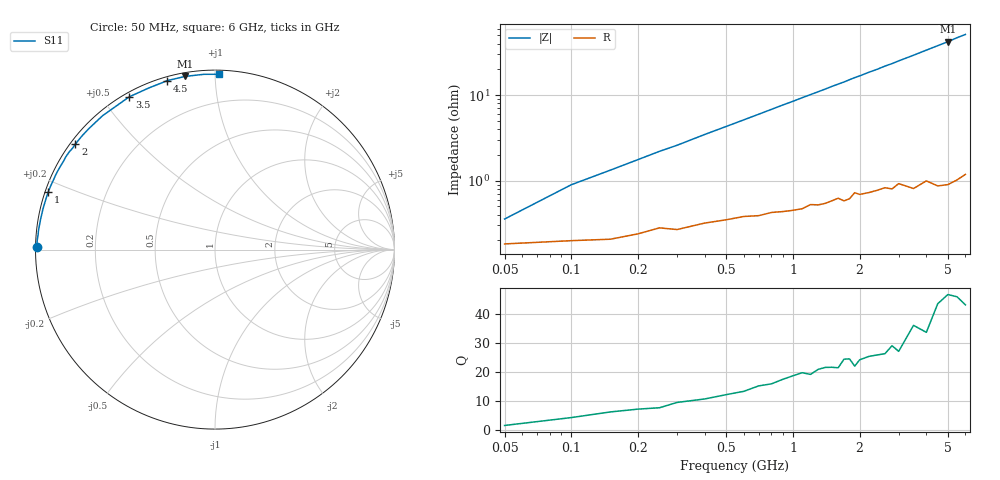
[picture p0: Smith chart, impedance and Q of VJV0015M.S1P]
! Infineon Technologies  Discrete & RF Semiconductors
! BB 914
! Si Tuning Diode in SOT23
! VR =
! S-Parameters:  July  1999
# GHz  S  MA  R  50
!  f  S11
! GHz  MAG  ANG
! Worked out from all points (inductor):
!   34 points, 50 MHz to 6 GHz, reference 50 ohm
!   read as one part to ground: L = 1.39 nH near 100 MHz
!   highest Q = 46.1 at 5 GHz (marker M1), where L = 1.34 nH
!   S11 on the Smith chart (normalised r, x): 50 MHz: 0.00, +0.01; 1 GHz: 0.01, +0.17; 2 GHz: 0.01, +0.34; 3.5 GHz: 0.02, +0.59; 4.5 GHz: 0.02, +0.76; 6 GHz: 0.02, +1.02
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0.05  0.9928 179.3
0.1  0.9921 178.0
0.25  0.9889 175.0
0.3  0.9894 174.1
0.5  0.9863 170.2
0.7  0.9848 166.4
0.8  0.9835 164.5
1  0.9827 160.8
1.1  0.9821 158.9
1.3  0.9804 155.3
1.4  0.9797 153.5
1.5  0.9784 151.6
1.6  0.977 149.9
1.7  0.9788 148.2
1.8  0.9778 146.3
1.9  0.9741 144.5
2  0.9755 142.9
2.2  0.9748 139.4
2.4  0.9738 136.3
2.6  0.9727 132.8
2.8  0.9741 129.9
3  0.971 126.6
3.5  0.9762 119.3
4  0.973 112.2
4.5  0.9782 105.7
5  0.9792 99.8
5.5  0.9786 93.6
6  0.9772 88.6
